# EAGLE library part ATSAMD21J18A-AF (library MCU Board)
MCU 32-Bit SAM D21J ARM Cortex M0+ RISC 256KB Flash 3.3V 64-Pin TQFP Tray
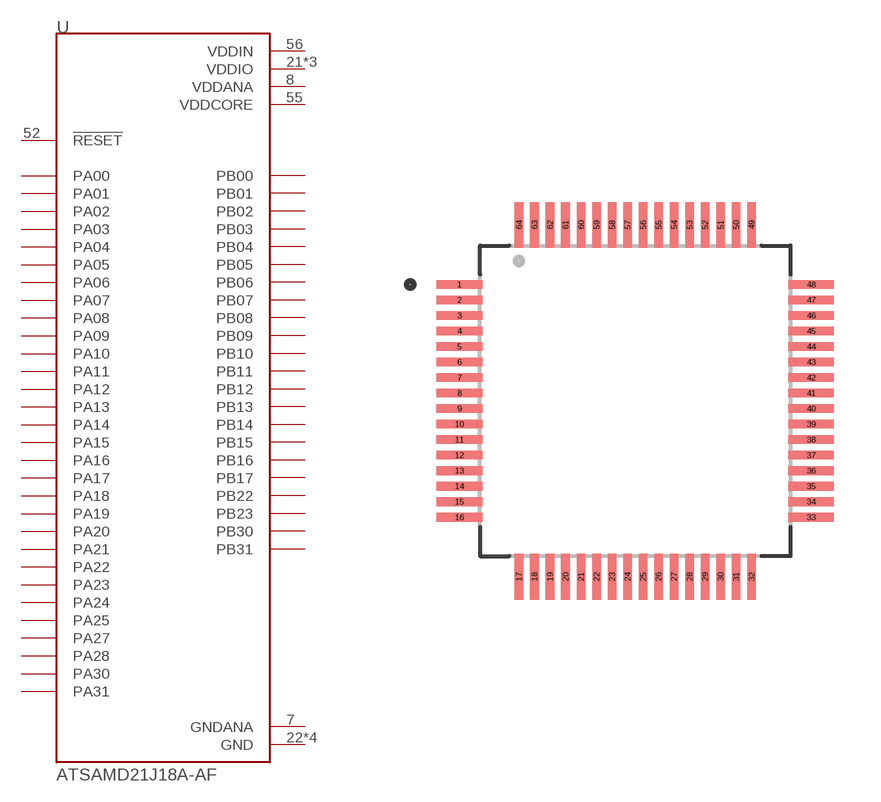
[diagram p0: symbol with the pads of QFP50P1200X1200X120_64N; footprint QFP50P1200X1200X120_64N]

Designator prefix U

## ATSAMD21J18A-AF (AVAILABILITY: Unavailable; DESCRIPTION: MCU 32-Bit SAM D21J ARM Cortex M0+ RISC 256KB Flash 3.3V 64-Pin TQFP Tray; MF: Microchip; MP: ATSAMD21J18A-AF; PACKAGE: TQFP-64 Microchip; PRICE: None)  [QFP50P1200X1200X120_64N]
1  PA00
2  PA01
3  PA02
4  PA03
5  PB04
6  PB05
7  GNDANA  pwr
8  VDDANA  pwr
9  PB06
10  PB07
11  PB08
12  PB09
13  PA04
14  PA05
15  PA06
16  PA07
17  PA08
18  PA09
19  PA10
20  PA11
21  VDDIO  pwr
22  GND  pwr
23  PB10
24  PB11
25  PB12
26  PB13
27  PB14
28  PB15
29  PA12
30  PA13
31  PA14
32  PA15
33  GND  pwr
34  VDDIO  pwr
35  PA16
36  PA17
37  PA18
38  PA19
39  PB16
40  PB17
41  PA20
42  PA21
43  PA22
44  PA23
45  PA24
46  PA25
47  GND  pwr
48  VDDIO  pwr
49  PB22
50  PB23
51  PA27
52  !RESET  in
53  PA28
54  GND  pwr
55  VDDCORE  pwr
56  VDDIN  pwr
57  PA30
58  PA31
59  PB30
60  PB31
61  PB00
62  PB01
63  PB02
64  PB03

## Footprint QFP50P1200X1200X120_64N (pad centres in mm)
smd 1.47 x 0.28: 1 -5.67,3.75; 2 -5.67,3.25; 3 -5.67,2.75; 4 -5.67,2.25; 5 -5.67,1.75; 6 -5.67,1.25; 7 -5.67,0.75; 8 -5.67,0.25; 9 -5.67,-0.25; 10 -5.67,-0.75; 11 -5.67,-1.25; 12 -5.67,-1.75; 13 -5.67,-2.25; 14 -5.67,-2.75; 15 -5.67,-3.25; 16 -5.67,-3.75; 33 5.67,-3.75; 34 5.67,-3.25; 35 5.67,-2.75; 36 5.67,-2.25; 37 5.67,-1.75; 38 5.67,-1.25; 39 5.67,-0.75; 40 5.67,-0.25; 41 5.67,0.25; 42 5.67,0.75; 43 5.67,1.25; 44 5.67,1.75; 45 5.67,2.25; 46 5.67,2.75; 47 5.67,3.25; 48 5.67,3.75
smd 0.28 x 1.47: 17 -3.75,-5.67; 18 -3.25,-5.67; 19 -2.75,-5.67; 20 -2.25,-5.67; 21 -1.75,-5.67; 22 -1.25,-5.67; 23 -0.75,-5.67; 24 -0.25,-5.67; 25 0.25,-5.67; 26 0.75,-5.67; 27 1.25,-5.67; 28 1.75,-5.67; 29 2.25,-5.67; 30 2.75,-5.67; 31 3.25,-5.67; 32 3.75,-5.67; 49 3.75,5.67; 50 3.25,5.67; 51 2.75,5.67; 52 2.25,5.67; 53 1.75,5.67; 54 1.25,5.67; 55 0.75,5.67; 56 0.25,5.67; 57 -0.25,5.67; 58 -0.75,5.67; 59 -1.25,5.67; 60 -1.75,5.67; 61 -2.25,5.67; 62 -2.75,5.67; 63 -3.25,5.67; 64 -3.75,5.67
